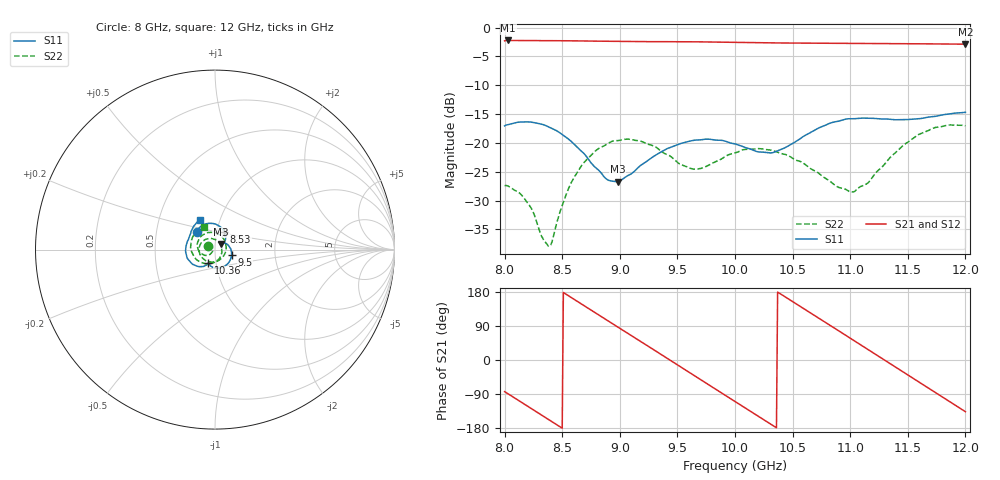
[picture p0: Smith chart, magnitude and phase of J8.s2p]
!Keysight Technologies,N5234A,MY52241180,A.10.60.03
!Date: Tuesday, May 30, 2023 15:26:48
!Correction: S11(Full 2 Port(1,2))
!S21(Full 2 Port(1,2))
!S12(Full 2 Port(1,2))
!S22(Full 2 Port(1,2))
!S2P File: Measurements: S11, S21, S12, S22:
# Hz S  dB  R 50
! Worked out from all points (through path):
!   401 points, 8 GHz to 12 GHz, reference 50 ohm
!   highest |S21| = -2.23 dB at 8.03 GHz (marker M1); lowest = -2.9 dB at 12 GHz (marker M2)
!   group delay of S21, straight-line fit = 536 ps
!   lowest |S11| = -26.7 dB at 8.98 GHz (marker M3), VSWR 1.10, Z = 53.4 + j3.38 ohm
!   |S11| at or under -10 dB: start of sweep to end of sweep
!   |S22| runs from -37.9 to -16.9 dB; largest |S21 - S12| = 0.0015
!   S11 on the Smith chart (normalised r, x): 8 GHz: 0.80, +0.16; 8.53 GHz: 1.08, +0.22; 9.5 GHz: 1.20, -0.07; 10.36 GHz: 0.92, -0.14; 12 GHz: 0.81, +0.27
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8e9  -17.05 136.4  -2.29 -83.5  -2.29 -83.5  -27.43 148.5
8.03e9  -16.83 133.3  -2.23 -89.2  -2.24 -89.2  -27.48 146.7
8.19e9  -16.35 112.8  -2.24 -120.0  -2.25 -120.1  -30.18 138.4
8.38e9  -17.20 84.5  -2.26 -156.7  -2.27 -156.8  -37.91 -178.7
8.53e9  -18.97 62.9  -2.28 174.2  -2.29 174.2  -29.18 -135.3
8.67e9  -21.49 45.7  -2.31 147.2  -2.32 147.1  -23.88 -149.8
8.98e9  -26.74 43.4  -2.40 87.5  -2.41 87.5  -19.60 156.8
9.15e9  -24.46 40.0  -2.42 54.8  -2.44 54.8  -19.58 122.8
9.34e9  -21.77 11.9  -2.44 18.3  -2.45 18.2  -21.13 77.8
9.5e9  -20.30 -16.5  -2.45 -12.6  -2.45 -12.7  -23.36 29.7
9.77e9  -19.35 -65.9  -2.49 -65.0  -2.50 -65.0  -23.88 -72.3
1e10  -20.17 -99.8  -2.56 -109.5  -2.57 -109.6  -21.73 -138.7
1.019e10  -21.50 -114.4  -2.61 -146.2  -2.62 -146.2  -21.00 -178.7
1.036e10  -21.45 -116.4  -2.66 -178.9  -2.66 -178.9  -21.54 149.7
1.067e10  -18.03 -130.6  -2.70 121.4  -2.71 121.4  -24.62 96.5
1.082e10  -16.61 -145.7  -2.71 92.5  -2.73 92.5  -26.58 65.9
1.097e10  -15.84 -162.3  -2.73 63.5  -2.74 63.5  -28.17 22.5
1.116e10  -15.71 178.1  -2.75 26.7  -2.75 26.6  -26.83 -45.3
1.134e10  -15.89 163.2  -2.76 -8.3  -2.77 -8.3  -22.69 -96.0
1.168e10  -15.52 142.4  -2.82 -74.3  -2.84 -74.3  -17.84 -171.5
1.183e10  -15.05 131.2  -2.85 -103.4  -2.86 -103.4  -16.98 155.9
1.2e10  -14.69 116.7  -2.87 -136.4  -2.88 -136.4  -17.05 116.2
